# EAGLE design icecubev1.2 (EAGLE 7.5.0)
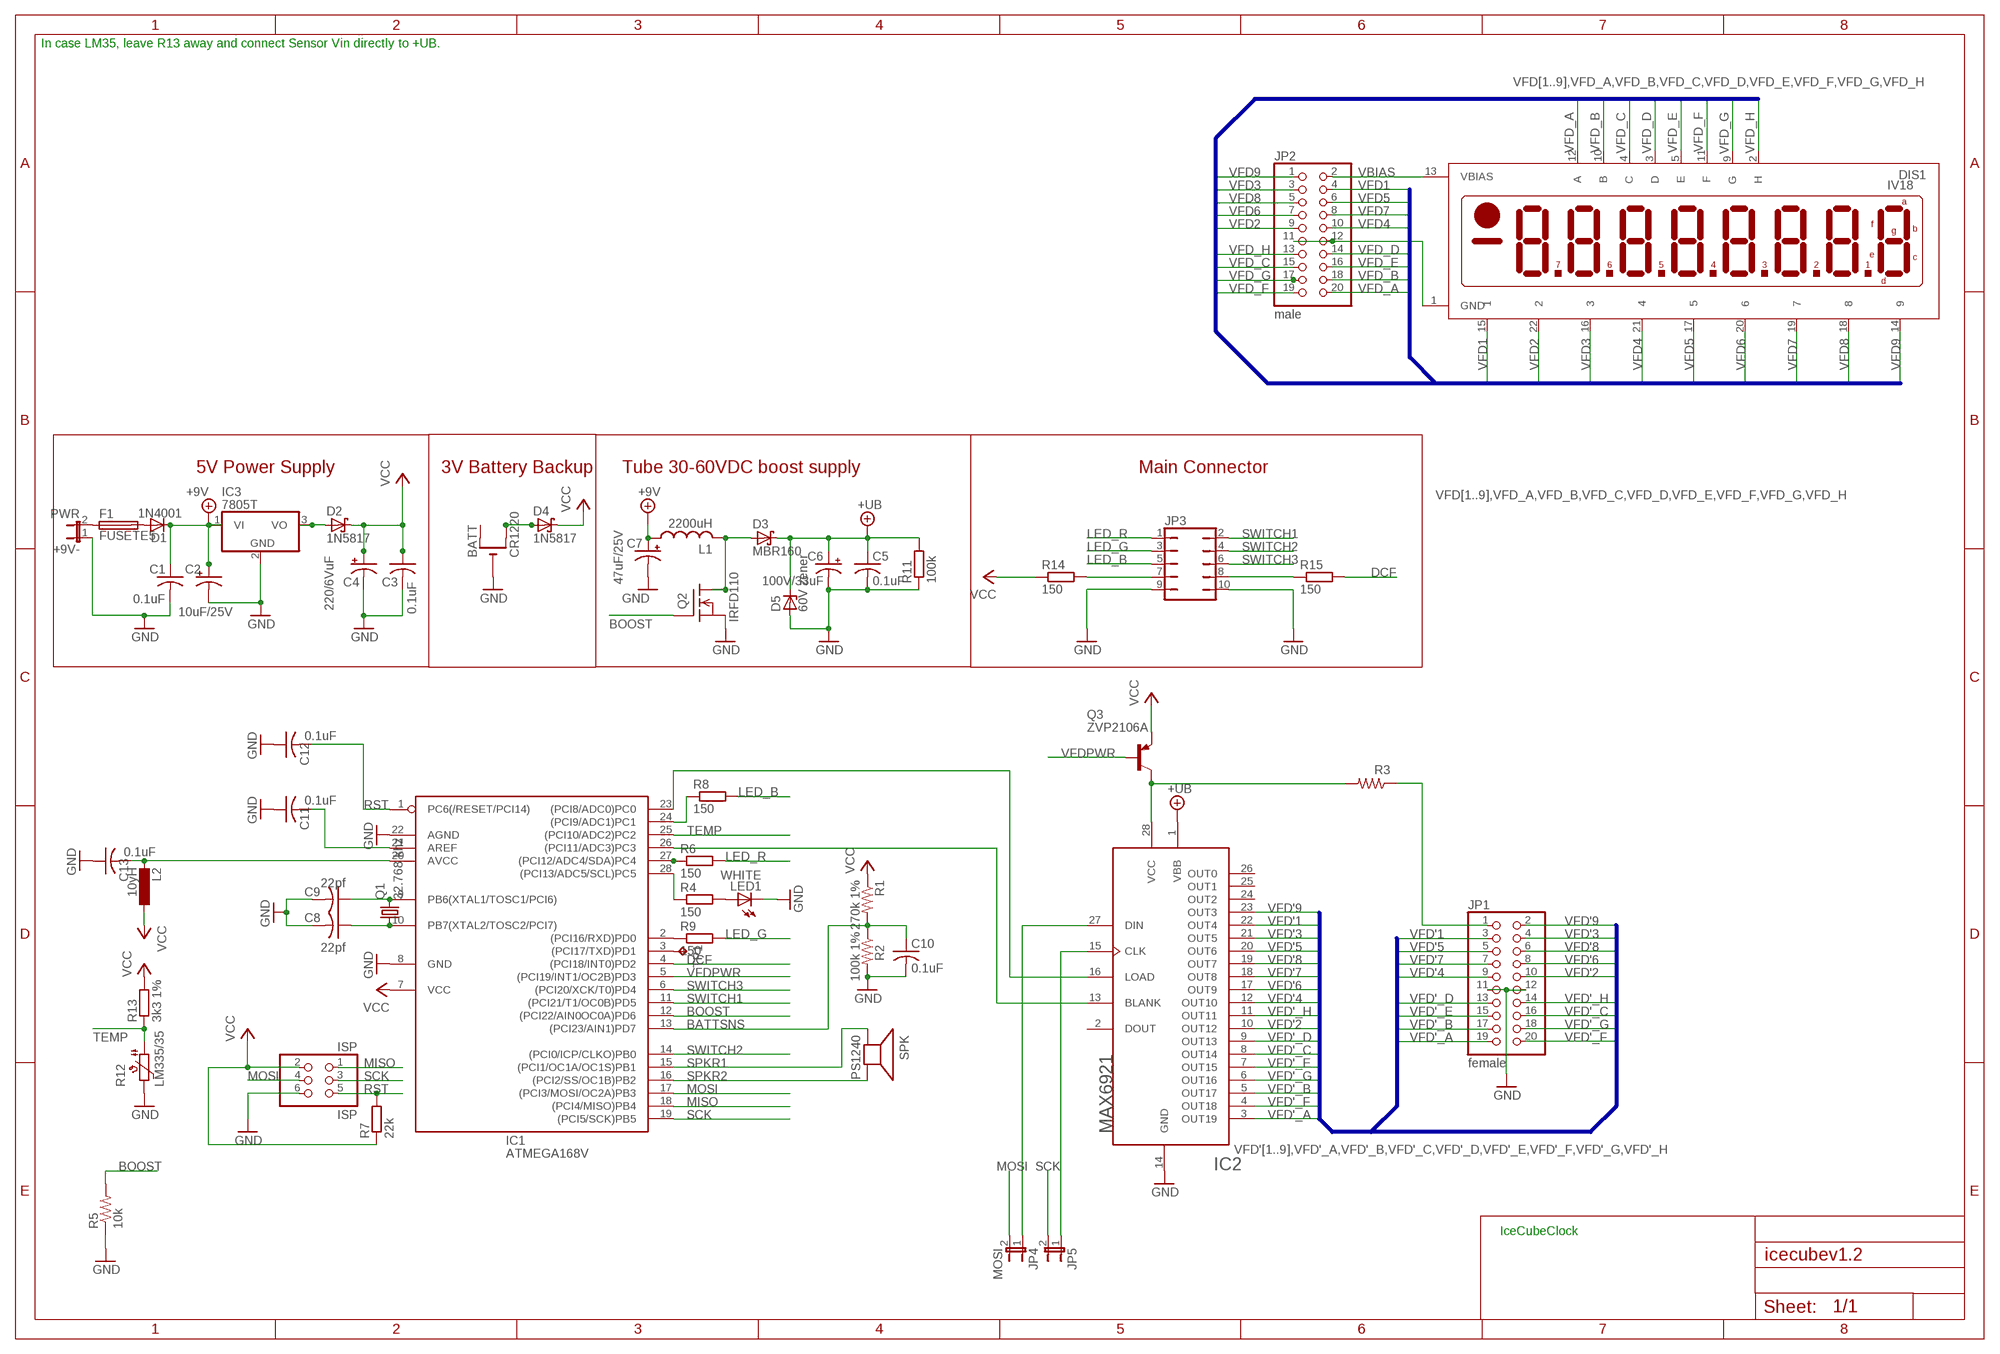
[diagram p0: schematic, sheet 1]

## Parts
+9V-  PWR  JP1E  [JP1]
BATT  CR1220  CR1220THM  [CR1220-THM]
C1  0.1uF  C-US025-025X050  [C025-025X050]
C2  10uF/25V  CPOL-USE2.5-6  [E2,5-6]
C3  0.1uF  C-US025-025X050  [C025-025X050]
C4  220/6VuF  CPOL-USE2.5-6  [E2,5-6]
C5  0.1uF  C-US025-024X044  [C025-024X044]
C6  100V/33uF  CPOL-USE3.5-8  [E3,5-8]
C7  47uF/25V  CPOL-USE2.5-6  [E2,5-6]
C8  22pf  C-US025-025X050  [C025-025X050]
C9  22pf  C-US025-025X050  [C025-025X050]
C10  0.1uF  C-US025-024X044  [C025-024X044]
C11  0.1uF  C-US025-025X050  [C025-025X050]
C12  0.1uF  C-US025-025X050  [C025-025X050]
C13  0.1uF  C-US025-025X050  [C025-025X050]
D1  1N4001  1N4004  [DO41-10]
D2  1N5817  SCHOTTKY-DIODEDO41  [DO41-10]
D3  MBR160  SCHOTTKY-DIODEDO41  [DO41-10]
D4  1N5817  SCHOTTKY-DIODEDO41  [DO41-10]
D5  60V zener  ZENER-DIODEDO41Z10  [DO41Z10]
DIS1  IV18  [IV18]
F1  FUSETE5  [TE5]
IC1  ATMEGA168V  ATMEGA168PROUND  [DIL28/3]
IC2  MAX6921  [PLCC-S28]
IC3  7805T  [TO220H]
ISP  ISP  PINHD-2X3  [2X03]
JP1  female  PINHD-2X10  [2X10]
JP2  male  PINHD-2X10  [2X10]
JP3  JP5Q  [JP5Q]
JP4  MOSI  JP1E  [JP1]
JP5  JP1E  [JP1]
L1  2200uH  L  [6000]
L2  10yH  L-EU0207/2V  [0207/2V]
LED1  WHITE  LED5MM  [LED5MM]
Q1  32.768 khz  CRYTALTC26V  [TC26V]
Q2  IRFD110  [DIL04]
Q3  ZVP2106A  BC327-16-PNP-TO92-EBC  [TO92-EBC]
R1  270k 1%  R-US_0207/10  [0207/10]
R2  100k 1%  R-US_0207/10  [0207/10]
R3  22  R-US_0207/5V  [0207/5V]
R4  150  R-EU_0204/5  [0204/5]
R5  10k  R-US_0207/5V  [0207/5V]
R6  150  R-EU_0204/5  [0204/5]
R7  22k  R-EU_0204/2V  [0204V@1]
R8  150  R-EU_0204/5  [0204/5]
R9  150  R-EU_0204/5  [0204/5]
R11  100k  R-EU_0204/2V  [0204V@1]
R12  LM335/35  PTC-SOD70  [SOD70]
R13  3k3 1%  R-EU_0204/5  [0204/5]
R14  150  R-EU_0204/5  [0204/5]
R15  150  R-EU_0204/2V  [0204V]
SPK  PS1240  SPEAKER/PS12  [PS12]
TP1  TPB2,54  [B2,54]

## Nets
+9V: C1.1 C2.+ C7.+ D1.C IC3.1(VI) L1.1
+UB: C5.1 C6.+ D3.C D5.C IC2.1(VBB) R11.2
BATTSNS: C10.1 IC1.13((PCI23/AIN1)PD7) R1.2 R2.1
BLANK: IC1.26((PCI11/ADC3)PC3) IC2.13(BLANK)
BOOST: IC1.12((PCI22/AIN0OC0A)PD6) Q2.3(G) R5.2
DCF: IC1.4((PCI18/INT0)PD2) R15.2
GND: +9V-.1 BATT.- C1.2 C2.- C3.2 C4.- C5.2 C6.- C7.- C8.2 C9.2 C10.2 C11.1 C12.1 C13.1 D5.A DIS1.1(GND) IC1.8(GND) IC1.22(AGND) IC2.14(GND) IC3.2(GND) ISP.6 JP1.11 JP1.12 JP2.11 JP2.12 JP3.9 JP3.10 LED1.K(C) Q2.4(S) R2.2 R5.1 R11.1 R12.2
LED_B: JP3.5 R8.2
LED_G: JP3.3 R9.2
LED_R: JP3.1 R6.2
LOAD: IC1.23((PCI8/ADC0)PC0) IC2.16(LOAD)
MISO: IC1.18((PCI4/MISO)PB4) ISP.1
MOSI: IC1.17((PCI3/MOSI/OC2A)PB3) ISP.4 JP4.2
N$1: C9.1 IC1.9(PB6(XTAL1/TOSC1/PCI6)) Q1.2
N$2: D3.A L1.2 Q2.1(D) Q2.2(D1)
N$3: C8.1 IC1.10(PB7(XTAL2/TOSC2/PCI7)) Q1.1
N$4: +9V-.2 F1.1
N$5: D1.A F1.2
N$6: IC1.27((PCI12/ADC4/SDA)PC4) R6.1
N$7: IC1.28((PCI13/ADC5/SCL)PC5) R4.1
N$8: IC1.24((PCI9/ADC1)PC1) R8.1
N$9: IC1.2((PCI16/RXD)PD0) R9.1
N$10: BATT.+2(+1) D4.A
N$11: JP3.8 R15.1
N$12: JP3.7 R14.2
N$13: LED1.A R4.2
N$14: C11.2 IC1.21(AREF)
N$15: C13.2 IC1.20(AVCC) L2.2
N$16: IC2.27(DIN) JP4.1
N$17: IC2.15(CLK) JP5.1
N$18: IC1.3((PCI17/TXD)PD1) TP1.TP
N$34: JP1.1 R3.1
N$39: IC2.28(VCC) Q3.C R3.2
N$53: D2.A IC3.3(VO)
RST: C12.2 IC1.1(PC6(/RESET/PCI14)) ISP.5 R7.2
SCK: IC1.19((PCI5/SCK)PB5) ISP.3 JP5.2
SPKR1: IC1.15((PCI1/OC1A/OC1S)PB1) SPK.P$1(+)
SPKR2: IC1.16((PCI2/SS/OC1B)PB2) SPK.P$2(-)
SWITCH1: IC1.11((PCI21/T1/OC0B)PD5) JP3.2
SWITCH2: IC1.14((PCI0/ICP/CLKO)PB0) JP3.4
SWITCH3: IC1.6((PCI20/XCK/T0)PD4) JP3.6
TEMP: IC1.25((PCI10/ADC2)PC2) R12.1 R13.1
VBIAS: DIS1.13(VBIAS) JP2.2
VCC: C3.1 C4.+ D2.C D4.C IC1.7(VCC) ISP.2 L2.1 Q3.E R1.1 R7.1 R13.2 R14.1
VFD1: DIS1.15 JP2.4
VFD2: DIS1.22 JP2.9
VFD3: DIS1.16 JP2.3
VFD4: DIS1.21 JP2.10
VFD5: DIS1.17 JP2.6
VFD6: DIS1.20 JP2.7
VFD7: DIS1.19 JP2.8
VFD8: DIS1.18 JP2.5
VFD9: DIS1.14 JP2.1
VFD'1: IC2.22(OUT4) JP1.3
VFD'2: IC2.10(OUT12) JP1.10
VFD'3: IC2.21(OUT5) JP1.4
VFD'4: IC2.12(OUT10) JP1.9
VFD'5: IC2.20(OUT6) JP1.5
VFD'6: IC2.17(OUT9) JP1.8
VFD'7: IC2.18(OUT8) JP1.7
VFD'8: IC2.19(OUT7) JP1.6
VFD'9: IC2.23(OUT3) JP1.2
VFD'_A: IC2.3(OUT19) JP1.19
VFD'_B: IC2.5(OUT17) JP1.17
VFD'_C: IC2.8(OUT14) JP1.16
VFD'_D: IC2.9(OUT13) JP1.13
VFD'_E: IC2.7(OUT15) JP1.15
VFD'_F: IC2.4(OUT18) JP1.20
VFD'_G: IC2.6(OUT16) JP1.18
VFD'_H: IC2.11(OUT11) JP1.14
VFD_A: DIS1.12(A) JP2.20
VFD_B: DIS1.10(B) JP2.18
VFD_C: DIS1.4(C) JP2.15
VFD_D: DIS1.3(D) JP2.14
VFD_E: DIS1.5(E) JP2.16
VFD_F: DIS1.11(F) JP2.19
VFD_G: DIS1.9(G) JP2.17
VFD_H: DIS1.2(H) JP2.13
VFDPWR: IC1.5((PCI19/INT1/OC2B)PD3) Q3.B
Unconnected: BATT.+1(+) IC2.2(DOUT) IC2.24(OUT2) IC2.25(OUT1) IC2.26(OUT0)

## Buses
VFD[1..9],VFD_A,VFD_B,VFD_C,VFD_D,VFD_E,VFD_F,VFD_G,VFD_H
VFD'[1..9],VFD'_A,VFD'_B,VFD'_C,VFD'_D,VFD'_E,VFD'_F,VFD'_G,VFD'_H

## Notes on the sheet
- In case LM35, leave R13 away and connect Sensor Vin directly to +UB.
- 5V Power Supply | 3V Battery Backup | Tube 30-60VDC boost supply | Main Connector
- IceCubeClock

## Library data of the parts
+9V- JP4 JP5 = jumper:JP1E: JUMPER
BATT = vfd:CR1220
C1 C3 C8 C9 C11-C13 = minimidi:C-US: CAPACITOR, American symbol
C2 C4 C7 = minimidi:CPOL-US: POLARIZED CAPACITOR, American symbol
C5 C10 = rcl-ez:C-US: CAPACITOR, American symbol
C6 = rcl-ez:CPOL-US: POLARIZED CAPACITOR, American symbol
D1 = minimidi:1N4004: DIODE
D2-D4 = usbbuck:SCHOTTKY-DIODE: Schottky Diode
D5 = diode:ZENER-DIODE: Z-Diode
DIS1 = vfd:IV18: LCD DISPLAY 8-character 7 segment
F1 = fuse:FUSE: Fuse
IC1 = avr:ATMEGA168*P: MICROCONTROLLER 16 kBytes FLASH 1 kBytes SRAM 512 Bytes EEPROM USART 8-channel 10 bit ADC
IC2 = vfd:MAX6921
IC3 = linear:78*: Positive VOLTAGE REGULATOR
ISP = pinhead-ez:PINHD-2X3: PIN HEADER
JP1 JP2 = pinhead:PINHD-2X10: PIN HEADER
JP3 = jumper:JP5Q: JUMPER
L1 = usbbuck:L
L2 = rcl:L-EU: INDUCTOR, European symbol
LED1 = led:LED: LED
Q1 = crystal:CRYTAL: CRYSTAL
Q2 = vfd:IRFD110
Q3 = transistor:*-PNP-: PNP Transistror
R1-R3 R5 = minimidi:R-US_: RESISTOR, American symbol
R4 R6 R8 R9 R13-R15 = resistor:R-EU_: RESISTOR, European symbol
R7 R11 = rcl:R-EU_: RESISTOR, European symbol
R12 = ptc-ntc:PTC-: Positive Temperature Coefficient Resistor (PTC) termistor; OC_FARNELL: unknown; OC_NEWARK: unknown
SPK = ybox2:SPEAKER: SPEAKER
TP1 = testpad:TP: Test pad

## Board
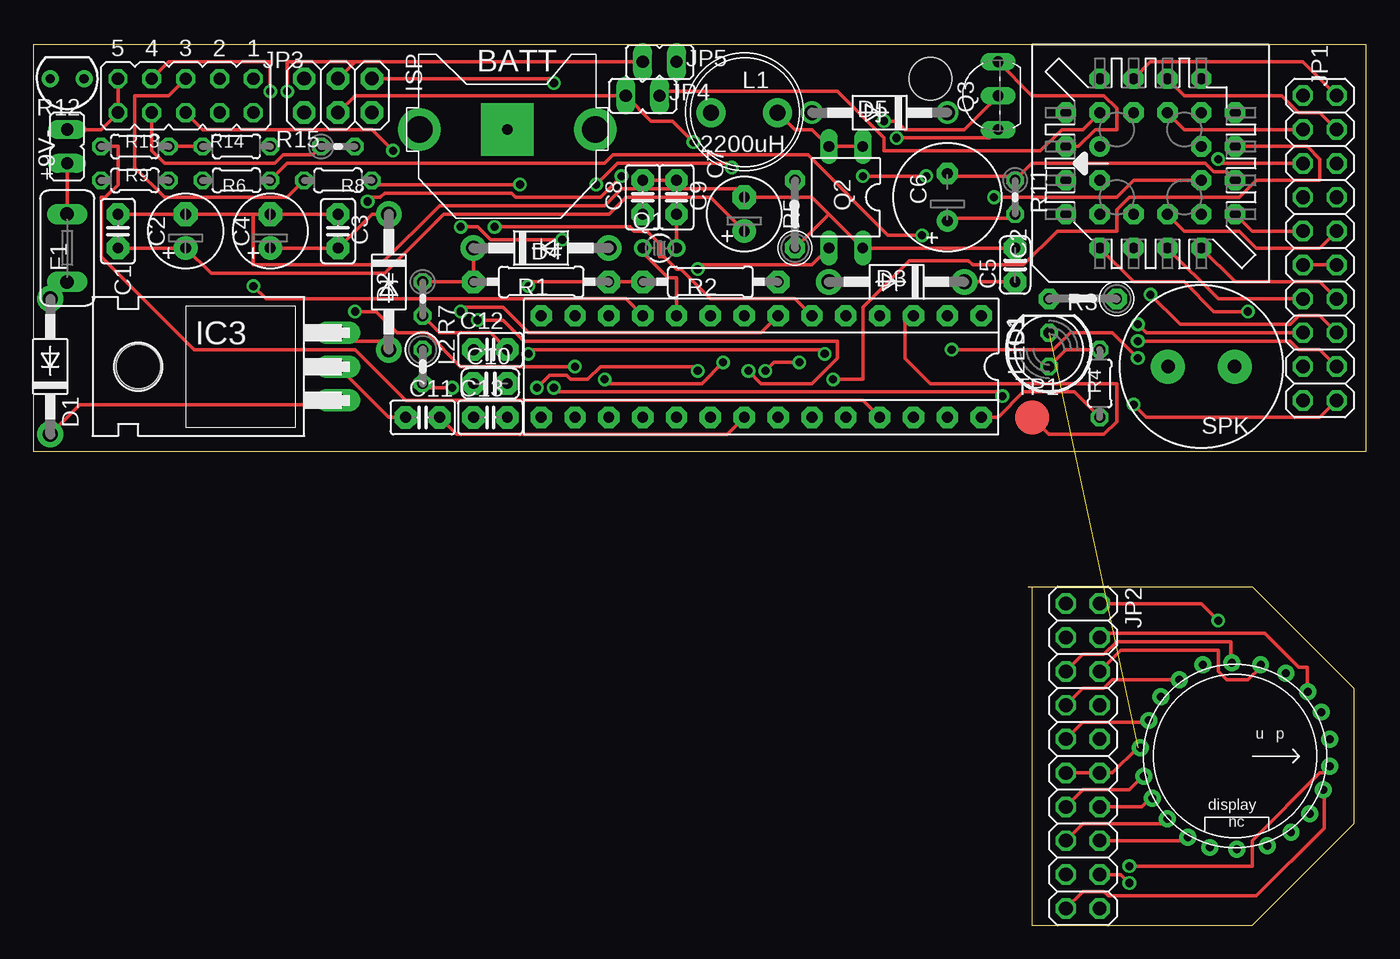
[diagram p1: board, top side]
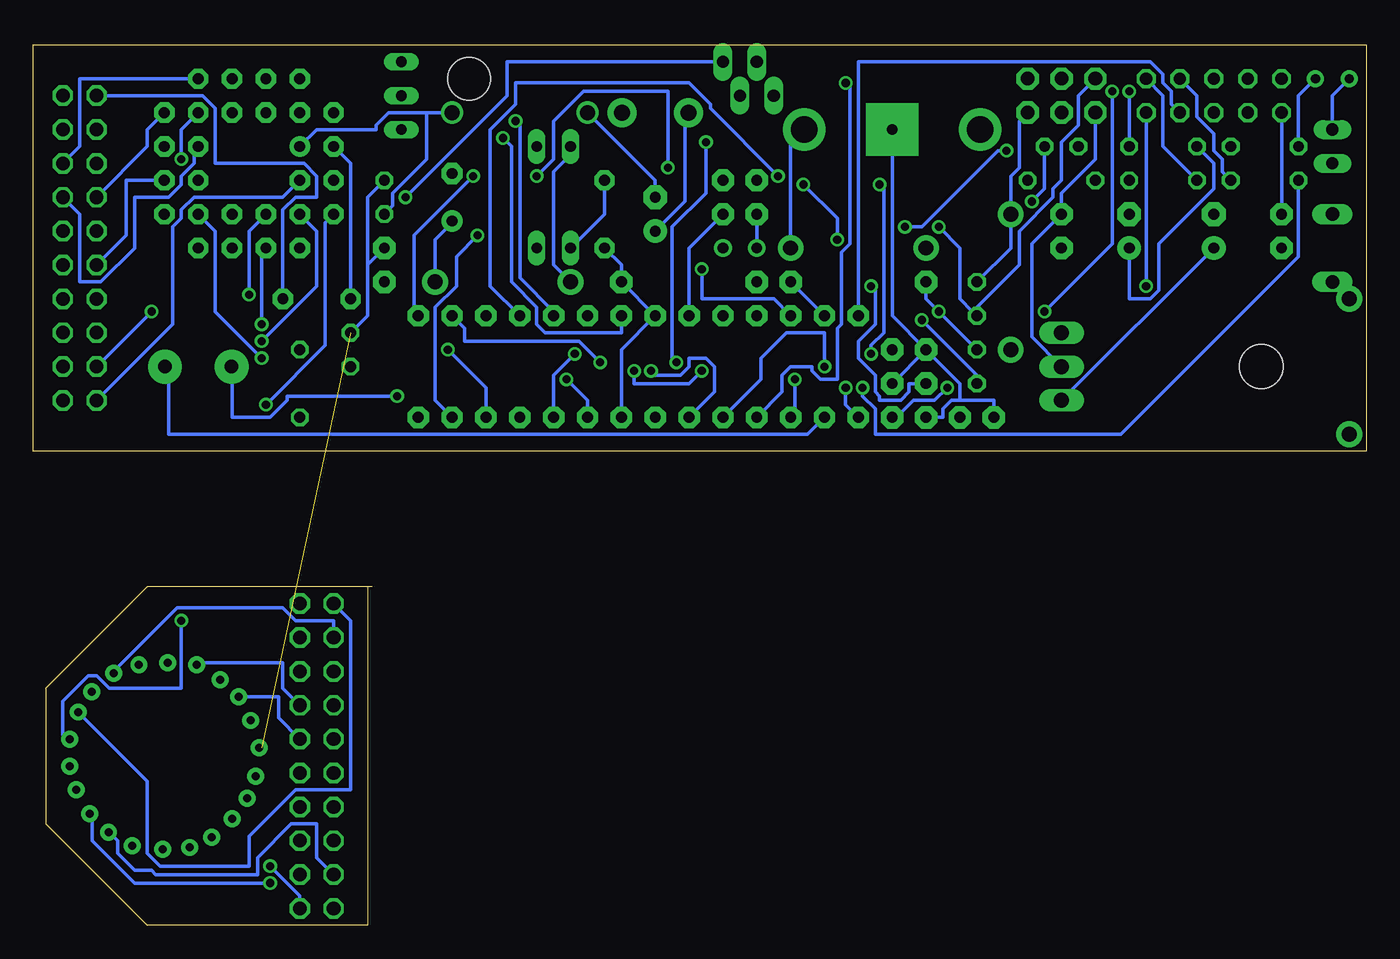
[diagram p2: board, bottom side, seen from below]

Size 100 x 66.03 mm. Coordinates in mm from the lower left corner, seen from the top.
Outline: 74.6,25.4 91.44,25.4 99.06,17.77 99.06,7.62
Outline: 74.93,25.39 74.93,0 91.44,0 99.06,7.61
Outline: 100,35.56 100,66.03 0,66.03 0,35.56 100,35.56
Copper layers (1*16): Top 0.035mm / dielectric 1.5mm / Bottom 0.035mm
Design rules "default": minimum track width 10mil, minimum drill 24mil, track to track 8mil, track to pad 8mil, pad to pad 8mil, via to via 8mil, smd to smd 8mil, copper to edge 40mil, drill to drill 8mil, minimum pad ring 10mil, minimum via ring 8mil, stop-mask expansion 4mil, vias tented up to drill 0mil, thermal gap 10mil
Holes 3.2 mm at 67.31,63.5

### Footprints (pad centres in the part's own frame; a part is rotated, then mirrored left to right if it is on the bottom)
JP1 = drill 0.914 long: 1 0,-1.27; 2 0,1.27
CR1220-THM = drill 2 pad 3.175: +1 -6.604,0; +2 6.604,0 | drill 0.8 pad 3.962 square: - 0,0
C025-025X050 = drill 0.813 pad 1.676 octagon: 1 -1.27,0; 2 1.27,0
E2,5-6 = drill 0.813 pad 1.778: + -1.27,0 | drill 0.813 pad 1.778 octagon: - 1.27,0
C025-024X044 = drill 0.813 pad 1.676 octagon: 1 -1.27,0; 2 1.27,0
E3,5-8 = drill 0.813 pad 1.6: + -1.778,0 | drill 0.813 pad 1.6 octagon: - 1.778,0
DO41-10 = drill 1.118 pad 1.93: A 5.08,0; C -5.08,0
DO41Z10 = drill 1.118: A 5.08,0; C -5.08,0
IV18 = drill 0.6 pad 1.27: 1 -0.635,-7.112; 2 1.524,-6.858; 3 3.175,-6.223; 4 4.699,-5.08; 5 6.096,-3.556; 6 6.858,-1.905; 7 6.985,0.127; 8 6.731,2.413; 9 5.715,4.191; 10 4.318,5.588; 11 2.54,6.604; 12 0.762,7.112; 13 -1.27,7.112; 14 -3.302,6.477; 15 -4.826,5.461; 16 -6.223,3.81; 17 -6.858,1.905; 18 -6.985,-0.254; 19 -6.858,-2.413; 20 -5.715,-4.191; 21 -4.445,-5.588; 22 -2.667,-6.477
TE5 = drill 1.016 long: 1 -2.54,0; 2 2.54,0
DIL28/3 = drill 0.813 pad 1.6 octagon: 1 -16.51,-3.81; 2 -13.97,-3.81; 3 -11.43,-3.81; 4 -8.89,-3.81; 5 -6.35,-3.81; 6 -3.81,-3.81; 7 -1.27,-3.81; 8 1.27,-3.81; 9 3.81,-3.81; 10 6.35,-3.81; 11 8.89,-3.81; 12 11.43,-3.81; 13 13.97,-3.81; 14 16.51,-3.81; 15 16.51,3.81; 16 13.97,3.81; 17 11.43,3.81; 18 8.89,3.81; 19 6.35,3.81; 20 3.81,3.81; 21 1.27,3.81; 22 -1.27,3.81; 23 -3.81,3.81; 24 -6.35,3.81; 25 -8.89,3.81; 26 -11.43,3.81; 27 -13.97,3.81; 28 -16.51,3.81
PLCC-S28 = drill 0.813 pad 1.524: 1 1.27,3.81 | drill 0.813 pad 1.524 octagon: 2 -1.27,6.35; 3 -1.27,3.81; 4 -3.81,6.35; 5 -6.35,3.81; 6 -3.81,3.81; 7 -6.35,1.27; 8 -3.81,1.27; 9 -6.35,-1.27; 10 -3.81,-1.27; 11 -6.35,-3.81; 12 -3.81,-6.35; 13 -3.81,-3.81; 14 -1.27,-6.35; 15 -1.27,-3.81; 16 1.27,-6.35; 17 1.27,-3.81; 18 3.81,-6.35; 19 6.35,-3.81; 20 3.81,-3.81; 21 6.35,-1.27; 22 3.81,-1.27; 23 6.35,1.27; 24 3.81,1.27; 25 6.35,3.81; 26 3.81,6.35; 27 3.81,3.81; 28 1.27,6.35
TO220H = drill 1.118 long: 1 -2.54,-10.16; 2 0,-10.16; 3 2.54,-10.16 | hole 3.302: 0,4.826
2X03 = drill 1.016 pad 1.676 octagon: 1 -2.54,-1.27; 2 -2.54,1.27; 3 0,-1.27; 4 0,1.27; 5 2.54,-1.27; 6 2.54,1.27
2X10 = drill 1.016 octagon: 1 -11.43,-1.27; 2 -11.43,1.27; 3 -8.89,-1.27; 4 -8.89,1.27; 5 -6.35,-1.27; 6 -6.35,1.27; 7 -3.81,-1.27; 8 -3.81,1.27; 9 -1.27,-1.27; 10 -1.27,1.27; 11 1.27,-1.27; 12 1.27,1.27; 13 3.81,-1.27; 14 3.81,1.27; 15 6.35,-1.27; 16 6.35,1.27; 17 8.89,-1.27; 18 8.89,1.27; 19 11.43,-1.27; 20 11.43,1.27
JP5Q = drill 0.914 octagon: 1 -5.08,-1.27; 2 -5.08,1.27; 3 -2.54,-1.27; 4 -2.54,1.27; 5 0,-1.27; 6 0,1.27; 7 2.54,-1.27; 8 2.54,1.27; 9 5.08,-1.27; 10 5.08,1.27
6000 = drill 1.2 pad 2.184: 1 -2.5,0; 2 2.5,0
0207/2V = drill 0.813 octagon: 1 -1.27,0; 2 1.27,0
LED5MM = drill 0.813 octagon: A -1.27,0; K 1.27,0
TC26V = drill 0.813: 1 -1.27,0; 2 1.27,0
DIL04 = drill 0.813 long: 1 -1.27,-3.81; 2 1.27,-3.81; 3 1.27,3.81; 4 -1.27,3.81
TO92-EBC = drill 0.813 long: B 0,-1.27; C 2.54,-1.27; E -2.54,-1.27
0207/10 = drill 0.813 pad 1.676 octagon: 1 -5.08,0; 2 5.08,0
0207/5V = drill 0.813 pad 1.524 octagon: 1 -2.54,0; 2 2.54,0
0204/5 = drill 0.813 octagon: 1 -2.54,0; 2 2.54,0
0204V@1 = drill 0.813 octagon: 1 -1.27,0; 2 1.27,0
SOD70 = drill 0.7 pad 1.27: 1 -1.27,0; 2 1.27,0
0204V = drill 0.813 octagon: 1 -1.27,0; 2 1.27,0
PS12 = drill 1 pad 2.54: P$1 -2.5,0; P$2 2.5,0
B2,54 = smd 2.54 x 2.54: TP 0,0

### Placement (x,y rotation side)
+9V-  2.54,58.42 180 top
BATT  35.56,59.69 0 top
C1  6.35,52.07 90 top
C2  11.43,52.07 90 top
C3  22.86,52.07 90 top
C4  17.78,52.07 90 top
C5  73.66,49.53 90 top
C6  68.58,54.61 90 top
C7  53.34,53.34 90 top
C8  45.72,54.61 90 top
C9  48.26,54.61 90 top
C10  34.29,40.64 0 top
C11  29.21,38.1 0 top
C12  34.29,43.18 0 top
C13  34.29,38.1 0 top
D1  1.27,41.91 90 top
D2  26.67,48.26 270 top
D3  64.77,48.26 180 top
D4  38.1,50.8 0 top
D5  63.5,60.96 180 top
DIS1  90.17,12.7 270 top
F1  2.54,50.8 270 top
IC1  54.61,41.91 180 top
IC2  83.82,57.15 90 top
IC3  12.7,41.91 90 top
ISP  22.86,62.23 180 top
JP1  96.52,50.8 270 top
JP2  78.74,12.7 270 top
JP3  11.43,62.23 180 top
JP4  45.72,62.23 90 top
JP5  46.99,64.77 90 top
L1  53.34,60.96 0 top
L2  29.21,41.91 270 top
LED1  76.2,43.18 90 top
Q1  46.99,50.8 0 top
Q2  60.96,54.61 180 top
Q3  71.12,62.23 90 top
R1  38.1,48.26 0 top
R2  50.8,48.26 0 top
R3  78.74,46.99 180 top
R4  80.01,40.64 90 top
R5  57.15,53.34 90 top
R6  15.24,55.88 180 top
R7  29.21,46.99 270 top
R8  22.86,55.88 180 top
R9  7.62,55.88 0 top
R11  73.66,54.61 270 top
R12  2.54,63.5 180 top
R13  7.62,58.42 0 top
R14  15.24,58.42 0 top
R15  22.86,58.42 0 top
SPK  87.63,41.91 0 top
TP1  74.93,38.1 0 top

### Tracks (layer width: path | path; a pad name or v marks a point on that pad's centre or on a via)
+9V
  Top 0.254: C1.1 C2.+ 13.34,48.89 26.35,48.89 30.8,53.34 43.18,53.34 44.45,54.61 50.8,54.61 C7.+ | D1.C 3.49,39.05 22.54,39.05 IC3.1
  Bottom 0.254: C7.+ 51.12,54.29 51.12,60.96 L1.1 | C2.+ IC3.1
+UB
  Top 0.254: R11.2 73.34,53.02 68.58,53.02 C6.+ | D3.C C5.1
  Bottom 0.254: D3.C 69.85,51.44 68.58,52.7 C6.+ | IC2.1 78.74,59.69 74.3,59.69 74.3,60.01 73.34,60.96 70.48,60.96 | D5.C 70.48,60.96 | R11.2 73.03,53.98 73.03,54.93 70.48,57.47 70.48,60.96
BATTSNS  (via drill 0.61)
  Top 0.254: v37.15,47.94 37.47,48.26 R1.2 R2.1
  Bottom 0.254: R1.2 IC1.13 | C10.1 34.29,40.64 34.29,40 34.92,39.37 36.51,39.37 36.51,39.69 36.83,40 36.83,41.28 38.1,42.55 38.1,43.81 36.83,45.08 36.83,47.62 v37.15,47.94
BLANK  (via drill 0.61)
  Top 0.254: v82.87,42.55 80.96,44.45 77.79,44.45 76.52,43.18 v68.9,43.18
  Bottom 0.254: IC2.13 86.36,52.07 86.36,46.04 v82.87,42.55 | v68.9,43.18 66.04,40.32 IC1.26
BOOST  (via drill 0.61)
  Top 0.254: v49.85,49.21 50.16,49.53 58.42,49.53 Q2.3
  Bottom 0.254: Q2.3 57.15,53.34 R5.2 | IC1.12 44.45,46.99 49.85,46.99 v49.85,49.21
DCF  (via drill 0.61)
  Top 0.254: v25.08,54.29 25.4,54.61 26.04,54.61 26.35,54.93 35.88,54.93 36.2,54.61 42.55,54.61 v44.13,56.2
  Bottom 0.254: R15.2 24.13,55.25 v25.08,54.29 | v44.13,56.2 49.21,61.28 49.21,61.59 50.8,63.18 63.82,63.18 63.82,61.59 65.72,59.69 65.72,47.94 IC1.4
GND  (1 unrouted)
  Top 0.254: JP3.9 JP3.10 5.08,59.69 +9V-.1 | C1.2 C2.- 16.51,53.34 | C3.2 C4.- 16.51,53.34 | IC3.2 26.67,38.1 C11.1 | C8.2 C9.2 48.9,55.25 | 59.69,53.34 58.42,54.61 C7.- 52.7,55.25 48.9,55.25 | 59.69,53.34 Q2.4 C5.2 | 59.69,53.34 R5.1 | JP1.12 JP1.11 | C6.- 68.58,56.2 73.34,56.2 R11.1 74.93,57.15 87.95,57.15 88.58,56.52 89.53,56.52 IC2.14 | 16.51,53.34 16.51,49.53 26.04,49.53 30.48,53.98 42.86,53.98 44.13,55.25 48.9,55.25 | DIS1.1 82.87,13.34 80.96,11.43 JP2.12 JP2.11
  Bottom 0.254: R12.2 2.54,62.23 +9V-.1 | ISP.6 20.32,57.47 22.86,54.93 C3.2 25.08,51.12 25.08,44.13 IC3.2 | C1.2 JP3.10 | C12.1 C10.2 | C13.1 31.75,38.1 31.75,38.73 31.11,39.37 30.48,39.37 | 30.48,39.37 27.94,39.37 C11.1 | C12.1 30.48,40.64 30.48,39.37 | BATT.- 35.56,45.72 C12.1 | R5.1 55.88,49.53 R2.2 IC1.8 55.88,43.18 IC1.22 | D5.A 53.34,55.88 C7.- | IC2.14 93.03,55.88 93.03,51.75 JP1.11 | LED1.K 74.93,45.72 74.93,49.53 | C5.2 74.93,49.53 | R11.1 74.93,54.61 74.93,49.53
LED_B
  Top 0.254: R8.2 19.05,54.61 9.84,54.61 7.62,56.83 7.62,62.23 10.16,62.23 JP3.5
LED_G
  Bottom 0.254: R9.2 10.79,56.52 10.79,57.47 11.43,58.1 11.43,59.37 12.7,60.64 12.7,62.23 JP3.3
LED_R
  Bottom 0.254: R6.2 15.24,58.42 15.24,62.23 JP3.1
LOAD  (via drill 0.61)
  Top 0.254: IC2.16 95.57,58.42 96.52,57.47 96.52,55.88 91.76,55.88 90.49,54.61 82.23,54.61 81.28,53.66 81.28,52.07 76.83,52.07 74.3,49.53 70.48,49.53 70.17,49.85 65.72,49.85 62.23,46.36 62.23,40.96 v60.01,40.96
  Bottom 0.254: v60.01,40.96 58.42,39.37 IC1.23
MISO  (via drill 0.61)
  Top 0.254: v39.05,63.18 38.73,63.5 ISP.1
  Bottom 0.254: IC1.18 43.81,40 43.81,41.28 43.18,41.91 41.59,41.91 41.59,41.59 40.96,40.96 39.69,40.96 39.69,44.77 39.37,45.08 39.37,50.48 38.73,51.12 38.73,62.87 v39.05,63.18
MOSI  (via drill 0.61)
  Top 0.254: ISP.4 24.13,62.23 JP4.2 46.35,60.33 47.94,60.33 v49.53,58.74 | v42.86,40.96 43.18,40.64 50.16,40.64 v51.75,42.23
  Bottom 0.254: IC1.17 42.86,38.42 v42.86,40.96 | v51.75,42.23 52.07,42.55 52.07,52.39 49.53,54.93 v49.53,58.74
N$1
  Top 0.254: C9.1 Q1.2
  Bottom 0.254: IC1.9 50.8,50.8 C9.1
N$2
  Top 0.254: Q2.1 Q2.2 58.42,59.69 57.15,59.69 55.88,60.96 L1.2
  Bottom 0.254: D3.A 60.96,49.53 60.96,56.52 59.69,57.78 Q2.2
N$3
  Top 0.254: IC1.10 48.26,48.58 47.62,48.58 45.72,50.48 Q1.1
  Bottom 0.254: C8.1 Q1.1
N$4
  Top 0.254: F1.1 +9V-.2
N$5
  Top 0.254: D1.A F1.2
N$6  (via drill 0.61)
  Top 0.254: R6.1 19.05,57.15 42.86,57.15 43.5,57.78 58.1,57.78 64.14,51.75 v66.67,51.75
  Bottom 0.254: v66.67,51.75 68.26,50.17 68.26,47.94 69.85,46.36 69.85,39.37 IC1.27
N$7
  Top 0.254: R4.1 78.11,40 74.3,40 72.39,38.1 IC1.28
N$8  (via drill 0.61)
  Top 0.254: R8.1 25.72,55.56 v36.51,55.56 | v37.15,42.86 37.47,43.18 59.05,43.18 v59.37,42.86
  Bottom 0.254: v36.51,55.56 36.2,55.25 36.2,44.45 37.15,43.5 v37.15,42.86 | v59.37,42.86 60.96,41.28 IC1.24
N$9  (via drill 0.61)
  Top 0.254: v37.78,40.32 38.73,41.28 40.01,41.28 40.32,40.96 41.59,40.96 42.55,41.91 49.53,41.91 v49.85,41.59 | v54.93,41.59 55.56,42.23 v57.47,42.23
  Bottom 0.254: R9.1 5.08,50.17 18.41,36.83 36.83,36.83 36.83,38.73 37.78,39.69 v37.78,40.32 | v49.85,41.59 50.8,40.64 54.93,40.64 v54.93,41.59 | v57.47,42.23 59.05,43.81 67.63,43.81 67.63,44.77 IC1.2
N$10
  Bottom 0.254: D4.A 43.18,58.74 42.23,59.69 BATT.+2
N$11
  Top 0.254: R15.1 20.95,57.78 18.73,57.78 18.1,57.15 9.84,57.15 8.89,58.1 JP3.8
N$12  (via drill 0.61)
  Top 0.254: v17.78,62.55 17.78,64.77 10.16,64.77 JP3.7
  Bottom 0.254: v17.78,62.55 R14.2
N$13
  Top 0.254: LED1.A 77.47,43.18 R4.2
N$14
  Top 0.254: IC1.21 52.07,36.83 31.75,36.83 C11.2
N$15  (via drill 0.61)
  Top 0.254: L2.2 29.53,40.32 v31.43,40.32 | v53.66,41.59 54.61,40.64 58.42,40.64 60.33,42.55 60.33,43.81 36.83,43.81 35.24,45.4 v33.34,45.4
  Bottom 0.254: v31.43,40.32 32.38,39.37 33.97,39.37 35.24,38.1 C13.2 | IC1.20 48.9,40 48.9,41.91 49.53,42.55 50.8,42.55 50.8,41.91 51.44,41.28 53.66,41.28 v53.66,41.59 | v33.34,45.4 29.21,41.28 L2.2
N$16
  Top 0.254: JP4.1 47.31,62.55 60.33,62.55 63.82,59.06 63.82,58.1 75.56,58.1 77.15,59.69 78.74,59.69 IC2.27
N$17  (via drill 0.61)
  Top 0.254: v72.07,54.61 81.28,54.61 82.55,55.88 IC2.15
  Bottom 0.254: JP5.1 64.45,64.77 64.45,62.23 v72.07,54.61
N$18
  Top 0.254: TP1.TP 76.2,36.83 80.33,36.83 81.28,37.78 81.28,40.64 67.31,40.64 65.41,42.55 65.41,45.72 IC1.3
N$34
  Bottom 0.254: R3.1 81.28,53.66 80.33,54.61 78.74,54.61 78.74,56.2 79.69,57.15 86.36,57.15 86.36,61.28 87.31,62.23 JP1.1
N$39
  Top 0.254: Q3.C 74.93,62.23 80.33,62.23 81.28,61.28 81.28,59.69 79.69,59.69 78.42,58.42 IC2.28
  Bottom 0.254: R3.2 76.2,57.15 IC2.28
N$53
  Top 0.254: IC3.3 23.5,43.81 26.04,43.81 D2.A
RST  (via drill 0.61)
  Top 0.254: R7.2 30.48,44.45 34.29,44.45 C12.2 | v62.23,56.2 v66.99,56.2 | v52.39,56.83 52.07,57.15 43.81,57.15 v42.23,55.56 | v39.69,51.44 34.29,51.44 33.34,52.39 v32.07,52.39
  Bottom 0.254: IC1.1 71.44,46.04 71.44,51.75 v66.99,56.2 | v62.23,56.2 60.96,57.47 60.96,60.33 58.74,62.55 52.39,62.55 v52.39,56.83 | v42.23,55.56 39.69,53.02 v39.69,51.44 | v32.07,52.39 30.48,50.8 30.48,46.99 29.53,46.04 | ISP.5 21.59,62.23 21.59,60.01 22.86,58.74 22.86,55.88 23.5,55.25 23.5,54.61 26.04,52.07 26.04,49.53 29.53,46.04 | 29.53,46.04 R7.2
SCK  (via drill 0.61)
  Top 0.254: 24.13,64.77 JP5.2 | ISP.3 24.13,64.77 | v40.64,41.91 32.07,41.91 29.53,44.45 27.3,44.45 25.72,46.04 v24.13,46.04 | v19.05,62.55 19.05,64.77 24.13,64.77
  Bottom 0.254: IC1.19 45.4,40.96 45.4,42.55 43.5,44.45 40.64,44.45 v40.64,41.91 | v24.13,46.04 19.05,51.12 v19.05,62.55
SPKR1  (via drill 0.61)
  Top 0.254: v39.05,40.32 39.37,40 72.39,40 v72.71,39.69
  Bottom 0.254: IC1.15 39.05,39.05 v39.05,40.32 | v72.71,39.69 80.96,39.69 80.96,39.37 82.23,38.1 85.09,38.1 85.09,41.91 SPK.P$1
SPKR2
  Bottom 0.254: IC1.16 41.91,36.83 89.85,36.83 89.85,41.91 SPK.P$2
SWITCH1  (via drill 0.61)
  Top 0.254: v16.51,47.94 17.46,46.99 44.45,46.99 IC1.11
  Bottom 0.254: v16.51,47.94 JP3.2
SWITCH2
  Bottom 0.254: JP3.4 14.61,61.59 14.61,62.55 15.24,63.18 15.24,63.82 16.19,64.77 38.1,64.77 IC1.14
SWITCH3  (via drill 0.61)
  Top 0.254: JP3.6 12.7,59.69 25.4,59.69 v26.99,58.1 | v34.61,52.39 44.77,52.39 45.09,52.07 46.04,52.07 46.99,51.12 46.99,50.17 47.31,50.17 48.26,49.21 48.58,49.21 50.8,46.99 57.15,46.99 IC1.6
  Bottom 0.254: v26.99,58.1 27.62,58.1 33.34,52.39 v34.61,52.39
TEMP
  Top 0.254: IC1.25 62.23,39.37 27.94,39.37 24.13,43.18 12.06,43.18 5.08,50.17 5.08,54.61 5.4,54.61 6.35,55.56 6.35,58.42 R13.1
  Bottom 0.254: R12.1 5.08,62.23 R13.1
VBIAS  (via drill 0.61)
  Top 0.254: v88.9,22.86 87.63,24.13 JP2.2
  Bottom 0.254: v88.9,22.86 88.9,17.78 94.3,17.78 95.25,18.73 95.89,18.73 97.79,16.83 97.79,14.29 97.47,13.97 DIS1.13
VCC  (via drill 0.61)
  Top 0.254: Q3.E 71.75,59.06 v64.77,59.06 | R14.1 R13.2 | R7.1 R1.1 D4.C | D2.C 25.4,53.34 C3.1 C4.+ | IC1.7 54.61,44.45 37.15,44.45 35.24,46.36 32.38,46.36 v32.07,46.04
  Bottom 0.254: v64.77,59.06 64.14,58.42 64.14,48.26 62.23,46.36 62.23,45.08 61.59,44.45 55.88,44.45 IC1.7 | R14.1 11.43,57.15 11.43,55.25 15.56,51.12 15.56,47.62 16.19,46.99 17.78,46.99 C4.+ | L2.1 v32.07,46.04 33.02,46.99 R1.1 | ISP.2 26.04,60.33 26.04,56.83 26.67,56.2 D2.C 26.67,50.8 R7.1
VFD1
  Top 0.254: JP2.4 80.33,21.91 92.39,21.91 94.93,19.37 95.57,19.37 95.57,17.78 DIS1.15
VFD2
  Top 0.254: JP2.9 78.74,15.24 83.5,15.24 DIS1.22
VFD3
  Bottom 0.254: JP2.3 77.47,22.86 80.33,22.86 81.28,23.81 89.22,23.81 93.98,19.05 DIS1.16
VFD4
  Bottom 0.254: DIS1.21 81.6,17.14 81.6,15.56 JP2.10
VFD5
  Top 0.254: JP2.6 81.6,20.64 88.9,20.64 88.9,19.05 89.53,18.41 91.12,18.41 92.08,19.37 DIS1.17
VFD6
  Top 0.254: DIS1.20 80.96,18.41 80.33,17.78 78.74,17.78 JP2.7
VFD7
  Bottom 0.254: JP2.8 81.28,17.78 81.28,19.68 87.63,19.68 DIS1.19
VFD8
  Top 0.254: JP2.5 78.74,20.32 80.33,20.32 81.28,21.27 89.85,21.27 89.85,19.68 DIS1.18
VFD9
  Bottom 0.254: DIS1.14 91.44,10.79 91.44,5.4 90.49,4.45 83.82,4.45 83.82,6.67 80.33,10.16 76.2,10.16 76.2,22.86 JP2.1
VFD'1
  Top 0.254: IC2.22 86.36,59.69 JP1.3
VFD'2
  Top 0.254: IC2.10 86.36,52.07 90.49,52.07 91.76,50.8 96.52,50.8 JP1.10
VFD'3
  Top 0.254: IC2.21 86.36,62.23 93.66,62.23 94.93,60.96 96.52,60.96 JP1.4
VFD'4
  Top 0.254: IC2.12 91.44,52.07 JP1.9
VFD'5  (via drill 0.61)
  Top 0.254: v88.9,57.47 89.22,57.15 JP1.5
  Bottom 0.254: IC2.20 88.9,59.69 v88.9,57.47
VFD'6
  Bottom 0.254: IC2.17 87.95,58.1 87.95,57.15 88.9,56.2 88.9,55.56 89.85,54.61 92.39,54.61 92.39,50.8 94.93,48.26 96.52,48.26 96.52,53.34 JP1.8
VFD'7
  Bottom 0.254: JP1.7 91.44,58.42 91.44,59.69 IC2.18
VFD'8
  Bottom 0.254: IC2.19 96.52,63.5 96.52,58.42 JP1.6
VFD'9
  Top 0.254: IC2.23 83.82,64.77 95.25,64.77 JP1.2
VFD'_A
  Bottom 0.254: JP1.19 89.53,45.08 89.53,52.39 88.9,53.02 88.9,53.66 87.95,54.61 81.28,54.61 IC2.3
VFD'_B  (via drill 0.61)
  Top 0.254: IC2.5 82.55,48.26 86.36,48.26 88.58,46.04 v91.12,46.04
  Bottom 0.254: JP1.17 v91.12,46.04
VFD'_C  (via drill 0.61)
  Top 0.254: v83.82,47.31 86.04,45.08 94.3,45.08 94.93,45.72 96.52,45.72 JP1.16
  Bottom 0.254: IC2.8 83.82,52.07 v83.82,47.31
VFD'_D
  Top 0.254: IC2.9 88.9,46.99 JP1.13
VFD'_E  (via drill 0.61)
  Top 0.254: v82.87,45.08 83.5,44.45 JP1.15
  Bottom 0.254: IC2.7 82.87,50.48 v82.87,45.08
VFD'_F  (via drill 0.61)
  Top 0.254: v82.55,39.05 83.5,38.1 96.52,38.1 JP1.20
  Bottom 0.254: IC2.4 78.11,52.7 78.11,43.5 v82.55,39.05
VFD'_G  (via drill 0.61)
  Top 0.254: v82.87,43.81 94.3,43.81 94.93,43.18 96.52,43.18 JP1.18
  Bottom 0.254: IC2.6 78.74,52.07 78.74,47.94 v82.87,43.81
VFD'_H
  Top 0.254: IC2.11 90.17,48.26 96.52,48.26 JP1.14
VFD_A  (via drill 0.61)
  Top 0.254: v82.23,4.45 91.44,4.45 91.44,6.35 96.52,11.43 96.84,11.43 97.16,11.75 DIS1.12
  Bottom 0.254: v82.23,4.45 80.01,2.22 JP2.20
VFD_B  (via drill 0.61)
  Top 0.254: v82.23,3.18 81.6,3.81 JP2.18
  Bottom 0.254: v82.23,3.18 92.39,3.18 95.57,6.35 95.57,8.25 DIS1.10
VFD_C
  Top 0.254: JP2.15 78.74,7.62 84.77,7.62 85.09,7.94 DIS1.4
VFD_D
  Top 0.254: JP2.14 83.19,8.89 83.82,9.52 DIS1.3
VFD_E
  Top 0.254: JP2.16 86.36,6.35 DIS1.5
VFD_F
  Top 0.254: JP2.19 78.74,2.54 80.33,2.54 80.64,2.22 91.76,2.22 96.84,7.3 96.84,10.16 DIS1.11
VFD_G
  Bottom 0.254: JP2.17 78.74,5.08 78.74,7.62 80.64,7.62 83.19,5.08 83.19,3.81 90.81,3.81 91.12,4.13 92.39,4.13 93.66,5.4 93.66,6.35 94.3,6.98 DIS1.9
VFD_H
  Top 0.254: JP2.13 78.74,10.16 82.23,10.16 83.19,11.11 DIS1.2
VFDPWR  (via drill 0.61)
  Top 0.254: Q3.B 69.85,59.69 65.41,59.69 64.77,60.33 v63.82,60.33
  Bottom 0.254: v63.82,60.33 63.5,60.01 63.5,48.58 60.96,46.04 IC1.5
